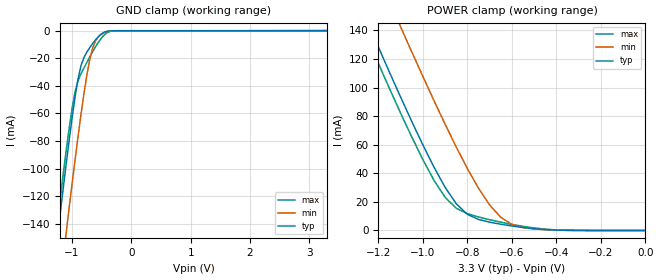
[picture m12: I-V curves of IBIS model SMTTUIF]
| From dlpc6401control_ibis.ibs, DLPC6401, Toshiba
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[Model]   SMTTUIF
Model_type   Input
Polarity   Non-Inverting
Vinl =   0.8000V
Vinh =   2.0000V
C_comp   1.443pF   NA   NA
|Variable   typ   min   max
[Voltage range]  3.3   3.0   3.6
[Temperature Range]   25.0000   125.000   0.000
[POWER Clamp Reference]   3.3000V   3.0000V   3.6000V
[GND Clamp Reference]   0.000V   0.000V   0.000V
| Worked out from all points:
|   GND clamp passes 1 mA (typ) near -0.45 V on its own axis
|   POWER clamp passes 1 mA (typ) near -0.48 V on its own axis
[GND_clamp]
| voltage   I(typ)   I(min)   I(max)
-3.3V     -944.9mA   -993.6mA   -933.7mA
-1.3V     -169.6mA   -220.5mA   -158.5mA
-1.25V    -151.2mA   -201.9mA   -140.2mA
-1.2V     -132.9mA   -183.4mA   -122.2mA
-1.1V     -97.22mA   -147mA     -87.5mA
-1V       -63.65mA   -111.4mA   -56.65mA
-900mV    -35.33mA   -77.27mA   -36.46mA
-800mV    -19.6mA    -45.94mA   -27.16mA
-700mV    -12.28mA   -20.75mA   -18.98mA
-600mV    -6.507mA   -7.188mA   -11.4mA
-450mV    -1.04mA    -1.222mA   -2.82mA
3.3V      2.124nA    35.56uA    -25.2uA
[POWER_clamp]
| voltage   I(typ)   I(min)   I(max)
-3.3V     917.5mA    964.8mA    906.4mA
-1.3V     164.1mA    213.9mA    152.5mA
-1.25V    146.1mA    195.8mA    134.5mA
-1.2V     128.2mA    177.9mA    116.7mA
-1.1V     93.14mA    142.3mA    81.93mA
-950mV    44.16mA    90.68mA    34.97mA
-850mV    18.6mA     58.27mA    15.49mA
-750mV    7.699mA    29.46mA    9.443mA
-650mV    4.358mA    9.175mA    5.797mA
-600mV    3.132mA    4.268mA    4.24mA
-500mV    1.241mA    1.079mA    1.758mA
0V        2.124nA    56.31nA    15.39nA
